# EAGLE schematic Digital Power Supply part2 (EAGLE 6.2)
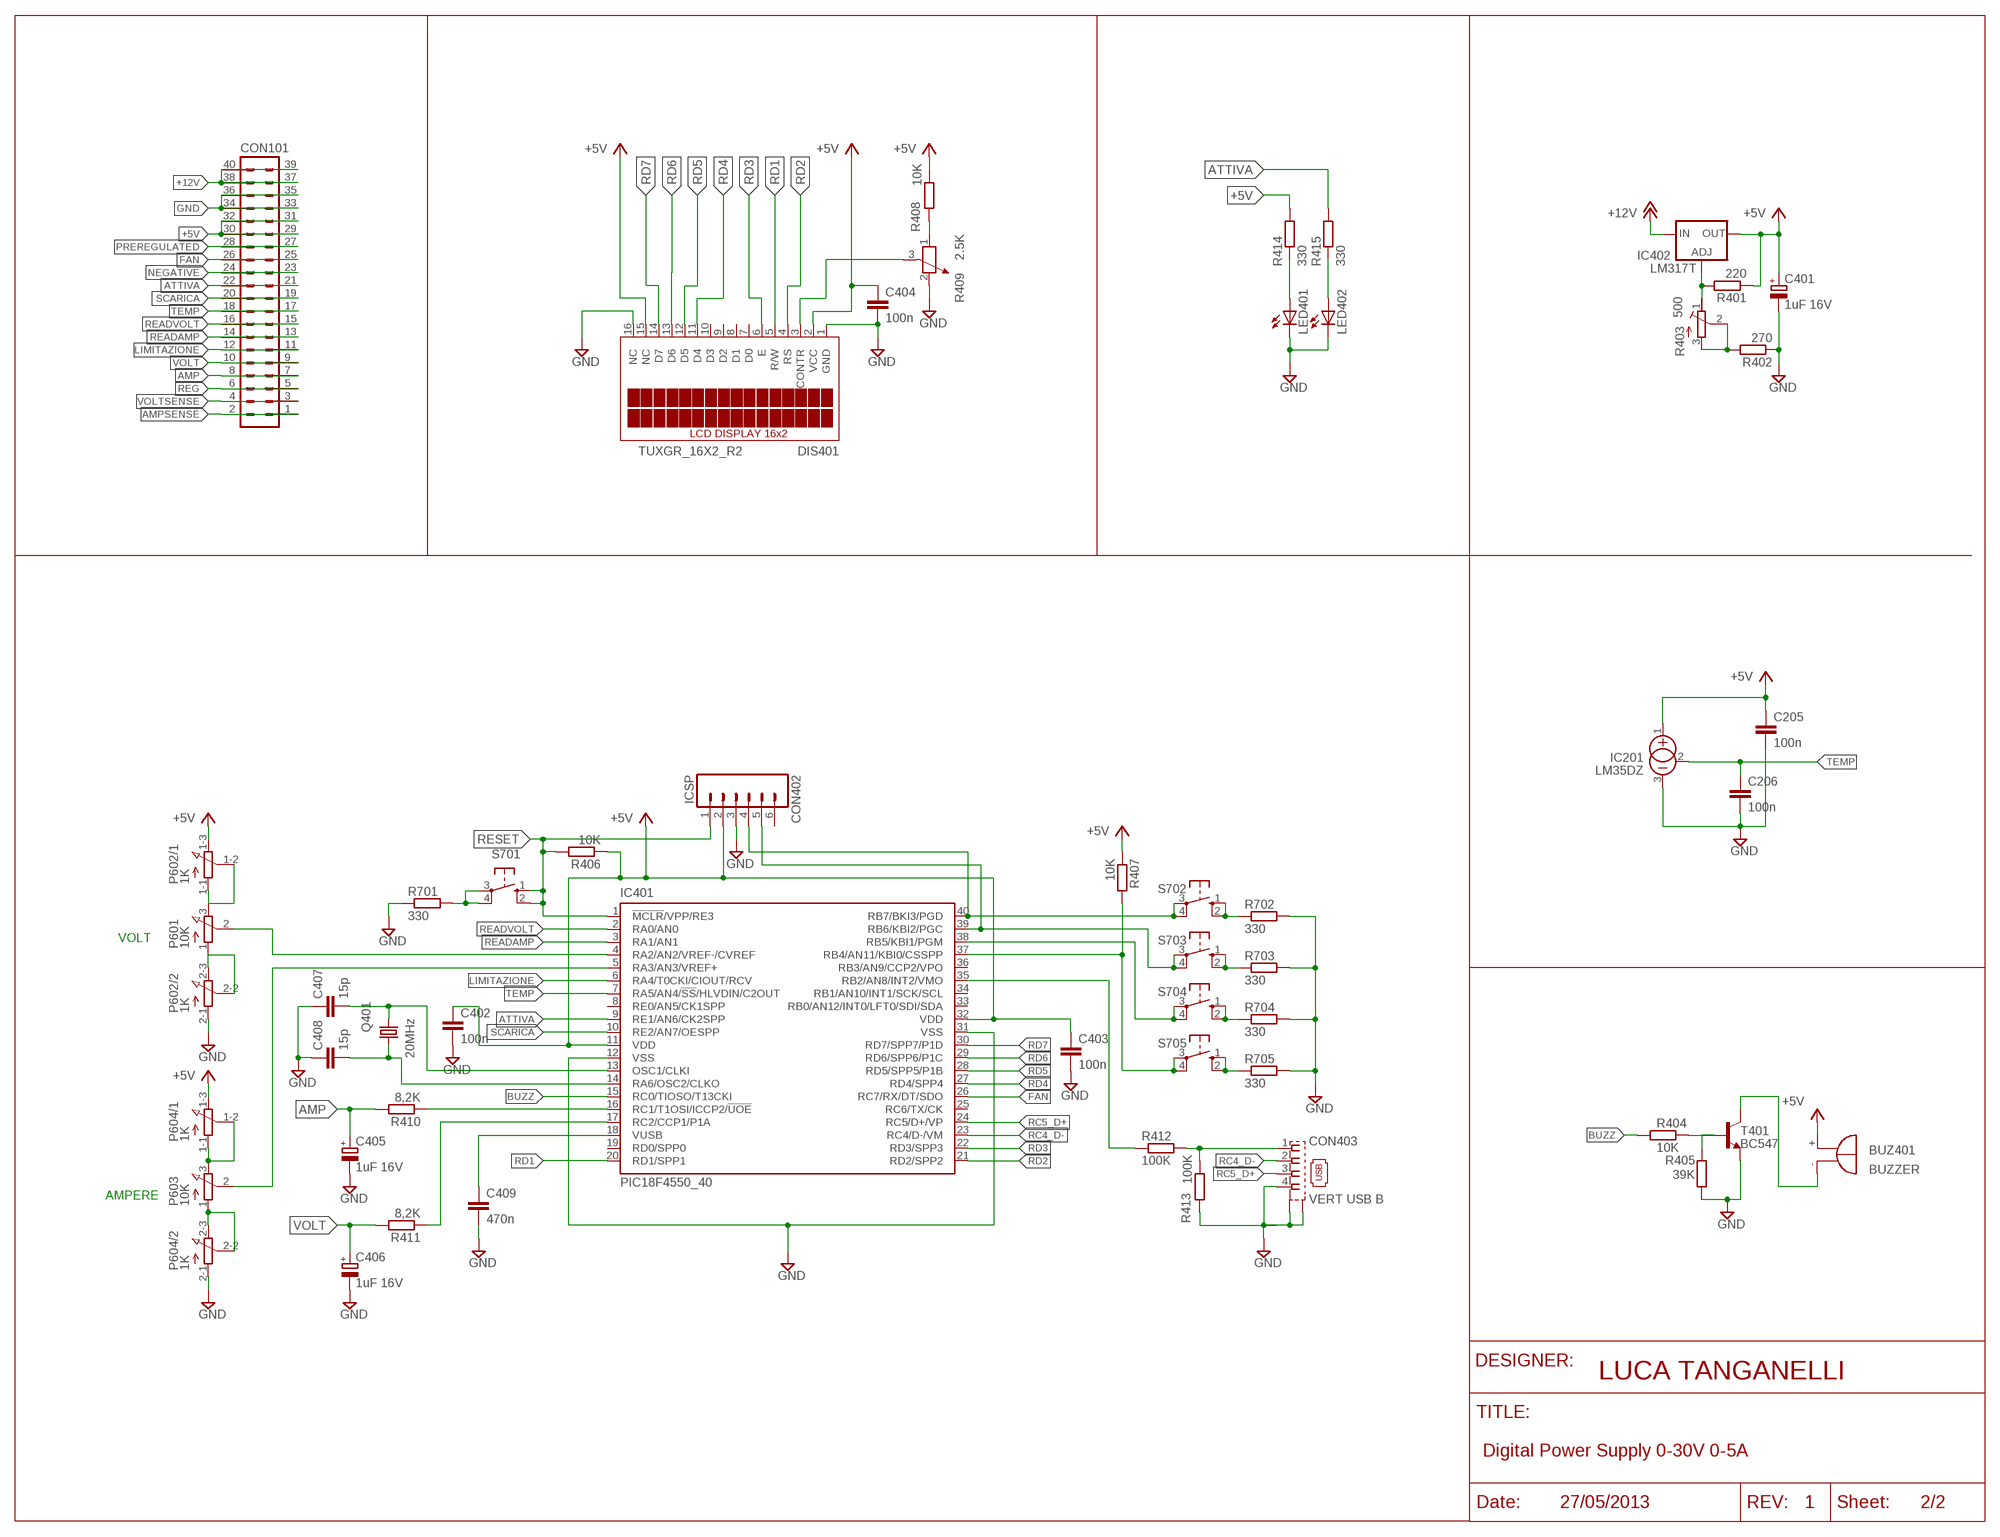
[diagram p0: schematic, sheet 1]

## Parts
BUZ401  BUZZER  F/HMB  [F/HMB]
C205  100n  C-EU050-024X044  [C050-024X044]
C206  100n  C-EU050-024X044  [C050-024X044]
C401  1uF 16V  CPOL-EUE2.5-5  [E2,5-5]
C402  100n  C-EU025-024X044  [C025-024X044]
C403  100n  C-EU025-024X044  [C025-024X044]
C404  100n  C-EU025-024X044  [C025-024X044]
C405  1uF 16V  CPOL-EUE2.5-5  [E2,5-5]
C406  1uF 16V  CPOL-EUE2.5-5  [E2,5-5]
C407  15p  C-EU025-024X044  [C025-024X044]
C408  15p  C-EU025-024X044  [C025-024X044]
C409  470n  C-EU025-024X044  [C025-024X044]
CON101  ML40  [ML40]
CON402  ICSP  MA06  [06PA]
CON403  VERT USB B  KUSBVX-BS1N  [KUSBVX-BS1N]
DIS401  TUXGR_16X2_R2  [TUXGR_16X2_R2]
IC201  LM35DZ  [TO-92]
IC401  PIC18F4550_40  [DIL40]
IC402  LM317T  LM317TS  [317TS]
LED401  LED3MM  [LED3MM]
LED402  LED3MM  [LED3MM]
P601  10K  3RP/1610N  [3RP/1610N]
P602  1K  3RP/1610G  [3RP/1610G]
P603  10K  3RP/1610N  [3RP/1610N]
P604  1K  3RP/1610G  [3RP/1610G]
Q401  20MHz  CRYSTALHC49S  [HC49/S]
R401  220  R-EU_0207/10  [0207/10]
R402  270  R-EU_0207/10  [0207/10]
R403  500  R-TRIMMT93YA  [RTRIMT93YA]
R404  10K  R-EU_0207/10  [0207/10]
R405  39K  R-EU_0207/10  [0207/10]
R406  10K  R-EU_0207/10  [0207/10]
R407  10K  R-EU_0207/10  [0207/10]
R408  10K  R-EU_0207/10  [0207/10]
R409  2.5K  POTENTIOMETER_PT-10  [PT-10]
R410  8,2K  R-EU_0207/10  [0207/10]
R411  8,2K  R-EU_0207/10  [0207/10]
R412  100K  R-EU_0207/10  [0207/10]
R413  100K  R-EU_0207/10  [0207/10]
R414  330  R-EU_0207/10  [0207/10]
R415  330  R-EU_0207/10  [0207/10]
R701  330  R-EU_0207/10  [0207/10]
R702  330  R-EU_0207/10  [0207/10]
R703  330  R-EU_0207/10  [0207/10]
R704  330  R-EU_0207/10  [0207/10]
R705  330  R-EU_0207/10  [0207/10]
S701  10-XX  [B3F-10XX]
S702  10-XX  [B3F-10XX]
S703  10-XX  [B3F-10XX]
S704  10-XX  [B3F-10XX]
S705  10-XX  [B3F-10XX]
T401  BC547  BC547-NPN-TO92-CBE  [TO92-CBE]

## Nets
+5V: BUZ401.+ C205.1 C401.+ C402.1 C403.1 C404.1 CON101.29 CON101.30 CON101.31 CON101.32 CON402.2 DIS401.2(VCC) DIS401.15(NC) IC201.1(+) IC401.11(VDD) IC401.32(VDD) IC402.2(OUT) P602.1-3(/1:E) P604.1-3(/1:E) R401.1 R406.1 R407.1 R408.1 R414.2
+12V: CON101.37 CON101.38 CON101.39 CON101.40 IC402.3(IN)
AMP: C405.+ CON101.7 CON101.8 R410.2
AMPSENSE: CON101.1 CON101.2
ATTIVA: CON101.21 CON101.22 IC401.9(RE1/AN6/CK2SPP) R415.2
BUZZ: IC401.15(RC0/TIOSO/T13CKI) R404.1
FAN: CON101.25 CON101.26 IC401.26(RC7/RX/DT/SDO)
GND: C205.2 C206.2 C401.- C402.2 C403.2 C404.2 C405.- C406.- C407.1 C408.1 C409.2 CON101.33 CON101.34 CON101.35 CON101.36 CON402.3 CON403.4 CON403.M1(S1) CON403.M2(S2) DIS401.1(GND) DIS401.16(NC) IC201.3(-) IC401.12(VSS) IC401.31(VSS) LED401.K(C) LED402.K(C) P602.2-1(/2:A) P604.2-1(/2:A) R402.1 R405.1 R409.2 R413.2 R701.1 R702.2 R703.2 R704.2 R705.2 T401.E
LIMITAZIONE: CON101.11 CON101.12 IC401.6(RA4/T0CKI/CIOUT/RCV)
N$1: IC401.35(RB2/AN8/INT2/VMO) R412.1
N$10: R705.1 S705.1(S) S705.2(S1)
N$11: IC401.37(RB4/AN11/KBI0/CSSPP) R407.2 S705.3(P) S705.4(P1)
N$32: R701.2 S701.3(P) S701.4(P1)
N$33: IC402.1(ADJ) R401.2 R403.1(A)
N$34: R402.2 R403.2(S) R403.3(E)
N$35: LED401.A R414.1
N$42: LED402.A R415.1
N$50: CON402.4 IC401.40(RB7/BKI3/PGD) S702.3(P) S702.4(P1)
N$60: CON402.5 IC401.39(RB6/KBI2/PGC) S703.3(P) S703.4(P1)
N$61: P601.1(A) P602.2-2(/2:S) P602.2-3(/2:E)
N$63: P601.3(E) P602.1-1(/1:A) P602.1-2(/1:S)
N$65: IC401.4(RA2/AN2/VREF-/CVREF) P601.2(S)
N$66: P603.1(A) P604.2-2(/2:S) P604.2-3(/2:E)
N$67: P603.3(E) P604.1-1(/1:A) P604.1-2(/1:S)
N$68: IC401.5(RA3/AN3/VREF+) P603.2(S)
N$69: IC401.16(RC1/T1OSI/ICCP2/!UOE) R410.1
N$70: IC401.17(RC2/CCP1/P1A) R411.1
N$72: DIS401.13(D6)
N$78: DIS401.3(CONTR) R409.3
N$82: CON403.1 R412.2 R413.1
N$83: C409.1 IC401.18(VUSB)
N$84: C408.2 IC401.14(RA6/OSC2/CLKO) Q401.1
N$85: C407.2 IC401.13(OSC1/CLKI) Q401.2
N$86: R704.1 S704.1(S) S704.2(S1)
N$87: R703.1 S703.1(S) S703.2(S1)
N$88: R702.1 S702.1(S) S702.2(S1)
N$89: R408.2 R409.1
N$90: IC401.38(RB5/KBI1/PGM) S704.3(P) S704.4(P1)
N$91: BUZ401.- T401.C
N$92: R404.2 R405.2 T401.B
NEGATIVE: CON101.23 CON101.24
PREREGULATED: CON101.27 CON101.28
RC4_D-: CON403.2 IC401.23(RC4/D-/VM)
RC5_D+: CON403.3 IC401.24(RC5/D+/VP)
RD1: DIS401.5(R/W) IC401.20(RD1/SPP1)
RD2: DIS401.4(RS) IC401.21(RD2/SPP2)
RD3: DIS401.6(E) IC401.22(RD3/SPP3)
RD4: DIS401.11(D4) IC401.27(RD4/SPP4)
RD5: DIS401.12(D5) IC401.28(RD5/SPP5/P1B)
RD6: IC401.29(RD6/SPP6/P1C)
RD7: DIS401.14(D7) IC401.30(RD7/SPP7/P1D)
READAMP: CON101.13 CON101.14 IC401.3(RA1/AN1)
READVOLT: CON101.15 CON101.16 IC401.2(RA0/AN0)
REG: CON101.5 CON101.6
RESET: CON402.1 IC401.1(!MCLR!/VPP/RE3) R406.2 S701.1(S) S701.2(S1)
SCARICA: CON101.19 CON101.20 IC401.10(RE2/AN7/OESPP)
TEMP: C206.1 CON101.17 CON101.18 IC201.2(CAN) IC401.7(RA5/AN4/!SS!/HLVDIN/C2OUT)
VOLT: C406.+ CON101.9 CON101.10 R411.2
VOLTSENSE: CON101.3 CON101.4
Unconnected: CON402.6 DIS401.7(D0) DIS401.8(D1) DIS401.9(D2) DIS401.10(D3) IC401.8(RE0/AN5/CK1SPP) IC401.19(RD0/SPP0) IC401.25(RC6/TX/CK) IC401.33(RB0/AN12/INT0/LFT0/SDI/SDA) IC401.34(RB1/AN10/INT1/SCK/SCL) IC401.36(RB3/AN9/CCP2/VPO)

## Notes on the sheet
- VOLT
- AMPERE
- LUCA TANGANELLI
- Digital Power Supply 0-30V 0-5A
- 27/05/2013 | 1 | 2/2

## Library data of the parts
BUZ401 = buzzer:F/HMB: BUZZER; OC_FARNELL: unknown; OC_NEWARK: unknown
C205 C206 C402-C404 C407-C409 = #-rcl:C-EU: CAPACITOR, European symbol
C401 C405 C406 = #-rcl:CPOL-EU: POLARIZED CAPACITOR, European symbol
CON101 = #-con-ml:ML40: HARTING; OC_FARNELL: unknown; OC_NEWARK: unknown
CON402 = #-con-amp-quick:MA06: AMP QUICK CONNECTOR; OC_FARNELL: unknown; OC_NEWARK: unknown
CON403 = #-con-kycon:KUSBVX-BS1N: USB B-type Receptacle Vertical, 4 Position, Through Hole Source: Sibalco Kycon KUSBVX-BS1N-xxx.pdf
DIS401 = #-display-lcd:TUXGR_16X2_R2: Tuxgraphics LCD display 16x2 characters reflective, without background light Source: tuxgr_12x2_r2.pdf; OC_FARNELL: unknown; OC_NEWARK: unknown
IC201 = #-linear:LM35DZ
IC401 = #-microchip:PIC18F4*_40: USB Microcontrollers with nanoWatt Technology High-Performance, Enhanced Flash, 28/40/44-Pin, Source: http://ww1.microchip.com/downloads/en/devicedoc/39632c.pdf; MF: MICROCHIP; MPN: PIC18F4550-I/P; OC_FARNELL: 9321357; OC_NEWARK: 74K8623
IC402 = #-v-reg:LM317TS: VOLTAGE REGULATOR
LED401 LED402 = #-led:LED: LED
P601 P603 = #-pot:3RP/1610N: 16mm Potentiometer one level Source: http://www.alphapotentiometers.net/html/16mm_pot_2.html
P602 P604 = #-pot:3RP/1610G: 16mm Potentiometer two level Source: http://www.alphapotentiometers.net/html/16mm_pot_2.html
Q401 = #-crystal:CRYSTAL: CRYSTAL; OC_FARNELL: 1667008; OC_NEWARK: unknown
R401 R402 R404-R408 R410-R415 R701-R705 = #-rcl:R-EU_: RESISTOR, European symbol
R403 = #-rcl:R-TRIMM: Trimm resistor
R409 = #-rcl:POTENTIOMETER_: Potentiometer
S701-S705 = #-switch-omron:10-XX: OMRON SWITCH; MPN: B3F-1000; OC_FARNELL: 176432; OC_NEWARK: 36M3542
T401 = #-transistor:*-NPN-: NPN Transistror BF959 corrected 2008.03.06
